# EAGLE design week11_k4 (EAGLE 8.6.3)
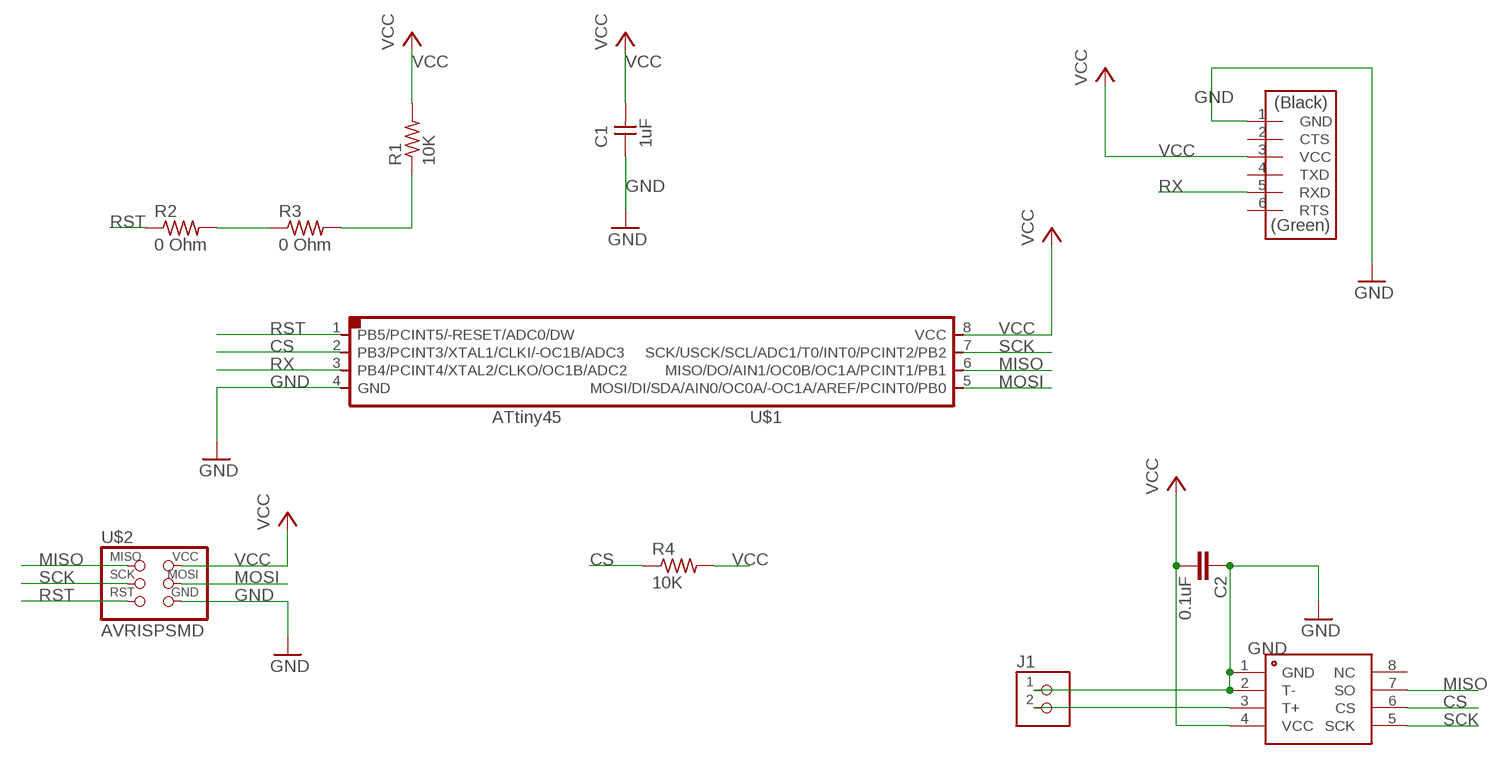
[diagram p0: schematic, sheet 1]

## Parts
C1  1uF  CAP-UNPOLARIZEDFAB  [C1206FAB]
C2  0.1uF  C-EUC0805K  [C0805K]
J1  TERM-1X02-ADAFRUIT  [3.5MMTERM]
MAX6675  MAX6675  [SO08]
R1  10K  RES-US1206FAB  [R1206FAB]
R2  0 Ohm  RES-US1206FAB  [R1206FAB]
R3  0 Ohm  RES-US1206FAB  [R1206FAB]
R4  10K  RES-US1206FAB  [R1206FAB]
U$1  ATTINY45SI  [SOIC8]
U$2  AVRISPSMD  [2X03SMD]
U$3  FTDI-SMD-HEADER  [1X06SMD]

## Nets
CS: MAX6675.6(CS) R4.1 U$1.2(PB3/PCINT3/XTAL1/CLKI/-OC1B/ADC3)
GND: C1.1 C2.1 J1.1 MAX6675.1(GND) MAX6675.2(T-) U$1.4(GND) U$2.6(GND) U$3.1(GND)
MISO: MAX6675.7(SO) U$1.6(MISO/DO/AIN1/OC0B/OC1A/PCINT1/PB1) U$2.1(MISO)
MOSI: U$1.5(MOSI/DI/SDA/AIN0/OC0A/-OC1A/AREF/PCINT0/PB0) U$2.4(MOSI)
N$1: J1.2 MAX6675.3(T+)
RST: R1.1 R2.1 R2.2 R3.1 R3.2 U$1.1(PB5/PCINT5/-RESET/ADC0/DW) U$2.5(RST)
RX: U$1.3(PB4/PCINT4/XTAL2/CLKO/OC1B/ADC2) U$3.5(RXD)
SCK: MAX6675.5(SCK) U$1.7(SCK/USCK/SCL/ADC1/T0/INT0/PCINT2/PB2) U$2.3(SCK)
VCC: C1.2 C2.2 MAX6675.4(VCC) R1.2 R4.2 U$1.8(VCC) U$2.2(VCC) U$3.3(VCC)
Unconnected: MAX6675.8(NC) U$3.2(CTS) U$3.4(TXD) U$3.6(RTS)

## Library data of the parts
C1 = fab:CAP-UNPOLARIZED
C2 = resistor:C-EU: CAPACITOR, European symbol
J1 = fab:TERM-1X02: 3.5mm terminal block, 2 positions ED555-2DS as found in the fablab inventory.
MAX6675 = maxim:MAX6675
R1-R4 = fab:RES-US: Resistor (US Symbol)
U$1 = fab:ATTINY45
U$2 = fab:AVRISP
U$3 = fab:FTDI-SMD-HEADER

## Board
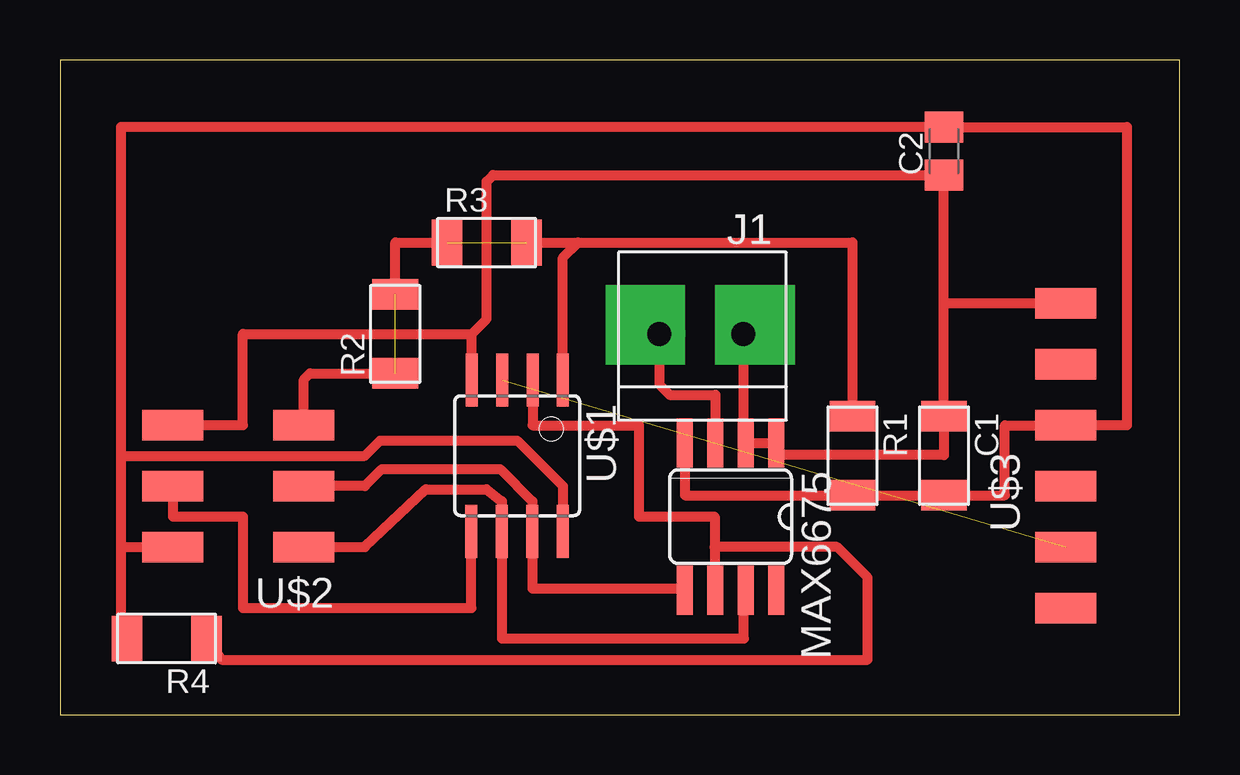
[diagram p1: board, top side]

Size 46.66 x 27.3 mm. Coordinates in mm from the lower left corner, seen from the top.
Outline: 0,0 46.66,0 46.66,27.3 0,27.3 0,0
Copper layers (1*16): Top 0.035mm / dielectric 1.5mm / Bottom 0.035mm
Design rules "default *": minimum track width 6mil, minimum drill 0.35mm, track to track 0.04mm, track to pad 0.04mm, pad to pad 0.04mm, via to via 0.04mm, smd to smd 0.04mm, copper to edge 40mil, drill to drill 6mil, minimum pad ring 10mil, minimum via ring 8mil, stop-mask expansion 4mil, vias tented up to drill 0mil, thermal gap 10mil

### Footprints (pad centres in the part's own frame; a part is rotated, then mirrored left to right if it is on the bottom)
C1206FAB = smd 1.27 x 1.905: 1 -1.651,0; 2 1.651,0
C0805K = smd 1.3 x 1.6: 1 -1,0; 2 1,0
3.5MMTERM = drill 1 pad 2.184: 1 1.8,0; 2 -1.7,0
SO08 = smd 0.66 x 2.032: 1 -1.905,-3.073; 2 -0.635,-3.073; 3 0.635,-3.073; 4 1.905,-3.073; 5 1.905,3.073; 6 0.635,3.073; 7 -0.635,3.073; 8 -1.905,3.073
R1206FAB = smd 1.27 x 1.905: 1 -1.651,0; 2 1.651,0
SOIC8 = smd 0.5 x 2.2: 1 -1.905,-3.154; 2 -0.645,-3.154; 3 0.625,-3.154; 4 1.895,-3.154; 5 1.905,3.154; 6 0.635,3.154; 7 -0.635,3.154; 8 -1.905,3.154
2X03SMD = smd 2.54 x 1.27: 1 -2.54,2.54; 2 2.92,2.54; 3 -2.54,0; 4 2.92,0; 5 -2.54,-2.54; 6 2.92,-2.54
1X06SMD = smd 2.54 x 1.27: 1 0,6.35; 2 0,3.81; 3 0,1.27; 4 0,-1.27; 5 0,-3.81; 6 0,-6.35

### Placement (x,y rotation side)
C1  36.83,10.79 270 top
C2  36.83,23.5 90 top
J1  26.67,15.88 0 top
MAX6675  27.94,8.26 180 top
R1  33.02,10.79 270 top
R2  13.97,15.88 90 top
R3  17.78,19.68 0 top
R4  4.45,3.17 180 top
U$1  19.05,10.79 180 top
U$2  7.62,9.53 180 top
U$3  41.91,10.79 0 top

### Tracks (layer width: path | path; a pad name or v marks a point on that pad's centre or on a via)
CS
  Top 0.152: 27.28,5.87 27.28,5.71 27.28,5.26 MAX6675.6 | 19.81,13.34 19.81,13.95 U$1.2
  Top 0.406: U$1.2 19.7,12.06 24.13,12.06 24.13,8.26 27.28,8.26 27.28,6.99 | 27.28,6.99 27.28,5.71 | R4.1 6.73,2.29 33.66,2.29 33.66,5.71 32.38,6.99 27.28,6.99
GND
  Top 0.152: 28.65,11.35 MAX6675.2 | 29.72,11.35 MAX6675.1 29.87,11.35 | 37.34,12.57 36.88,12.57 C1.1 36.74,12.42 36.73,12.42 | 4.72,12.12 U$2.6 | 17.07,13.95 U$1.4
  Top 0.406: 36.74,12.42 36.83,12.42 36.83,10.82 29.72,10.82 29.72,11.35 | C1.1 36.83,17.14 | U$1.4 17.16,15.88 | 4.72,12.12 4.72,12.06 7.62,12.06 7.62,15.88 17.16,15.88 | MAX6675.1 MAX6675.2 28.47,11.43 J1.1 | 17.16,15.88 17.78,16.5 17.78,22.23 18.05,22.5 C2.1 36.83,17.14 | U$3.1 36.83,17.14
MISO
  Top 0.152: 28.5,4.65 28.5,5.11 MAX6675.7 | 18.44,7.09 18.44,7.54 U$1.6 | 10.21,7.09 U$2.1
  Top 0.406: 28.5,4.65 28.5,3.17 18.41,3.17 U$1.6 18.41,8.89 17.78,9.4 15.24,9.4 12.7,6.99 U$2.1
MOSI
  Top 0.406: U$2.4 4.7,8.26 7.62,8.26 7.62,4.45 17.14,4.45 U$1.5
N$1
  Top 0.406: J1.2 24.97,13.77 25.4,13.34 27.3,13.34 MAX6675.3
N$2  (via drill 0 pad 3.3)
  other vias: 24.38,16.26
N$3  (via drill 0 pad 3.3)
  other vias: 28.96,16.26
RST  (2 unrouted)
  Top 0.152: 21.03,13.95 U$1.1
  Top 0.406: R2.2 13.97,19.68 R3.1 | R3.2 21.59,19.68 | 21.59,19.68 33.02,19.68 R1.1 | U$1.1 20.95,19.05 21.59,19.68 | U$2.5 10.16,13.97 10.41,14.22 R2.1
RX  (1 unrouted)
SCK
  Top 0.152: 19.81,7.09 19.81,7.54 U$1.7 | 25.91,5.26 MAX6675.5
  Top 0.406: U$2.3 12.7,9.53 13.41,10.24 18.34,10.24 19.68,8.89 U$1.7 19.68,5.26 25.91,5.26
VCC
  Top 0.152: 33.07,9.22 R1.2 32.92,9.22 | 36.73,9.22 C1.2 36.88,9.22 | 26.06,10.9 26.06,11.2 MAX6675.4 | 41.91,12.12 U$3.3 41.91,11.96
  Top 0.406: MAX6675.4 26.04,9.14 R1.2 36.88,9.14 36.88,9.22 | C1.2 39.37,9.14 39.37,12.06 U$3.3 44.45,12.06 44.45,24.5 C2.2 2.54,24.5 2.54,10.79 | 2.54,10.79 2.54,6.99 | 2.54,6.99 U$2.2 | 2.54,10.79 12.7,10.79 13.34,11.43 19.05,11.43 20.95,9.53 U$1.8 | 2.54,6.99 2.54,3.43 R4.2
